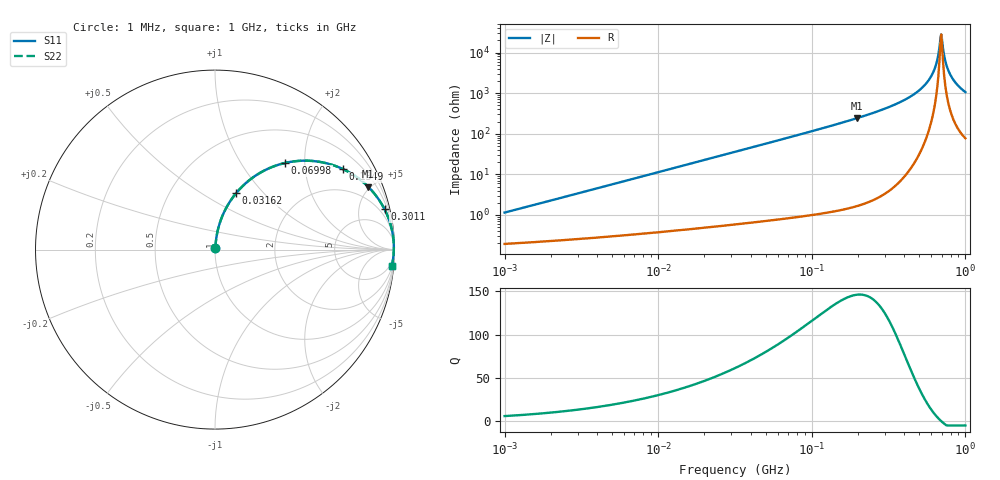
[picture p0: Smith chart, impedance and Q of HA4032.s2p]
# MHz S MA R 50
!Freq  MagS11  AngS11  MagS21  AngS21  MagS12  AngS12  MagS22  AngS22
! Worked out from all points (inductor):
!   801 points, 1 MHz to 1 GHz, reference 50 ohm
!   read as one part in series: L = 180 nH near 1.035 MHz
!   highest Q = 146 at 197.2 MHz (marker M1), where L = 196 nH
!   self-resonance near 689.8 MHz
!   S11 on the Smith chart (normalised r, x): 1 MHz: 1.00, +0.02; 31.62 MHz: 1.01, +0.72; 69.98 MHz: 1.02, +1.60; 134.9 MHz: 1.02, +3.17; 301.1 MHz: 1.07, +8.38; 1 GHz: 3, -21
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1  0.01145 79.6  0.998 -0.6  0.998 -0.6  0.01145 79.6
3.180534  0.03595 83.8  0.9968 -2.1  0.9968 -2.1  0.03595 83.8
10.02882  0.1124 81.7  0.99 -6.4  0.99 -6.4  0.1124 81.7
31.62278  0.3357 69.5  0.9365 -19.6  0.9365 -19.6  0.3357 69.5
31.89701  0.3383 69.3  0.9356 -19.8  0.9356 -19.8  0.3383 69.3
69.9842  0.6214 51.0  0.7771 -38.4  0.7771 -38.4  0.6214 51.0
100.5773  0.7547 40.5  0.6496 -49.0  0.6496 -49.0  0.7547 40.5
134.8963  0.8429 32.1  0.5317 -57.4  0.5317 -57.4  0.8429 32.1
197.2423  0.9223 22.3  0.3802 -67.3  0.3802 -67.3  0.9223 22.3
301.1272  0.9709 13.4  0.2316 -76.1  0.2316 -76.1  0.9709 13.4
317.1393  0.9747 12.4  0.2152 -77.1  0.2152 -77.1  0.9747 12.4
444.1197  0.9911 6.7  0.1169 -82.3  0.1169 -82.3  0.9911 6.7
555.9043  0.9958 3.3  0.05727 -84.2  0.05727 -84.2  0.9958 3.3
627.3357  0.9966 1.5  0.02639 -81.9  0.02639 -81.9  0.9966 1.5
649.3816  0.9966 1.0  0.01772 -78.6  0.01772 -78.6  0.9966 1.0
678.0317  0.9965 0.4  0.007339 -61.7  0.007339 -61.7  0.9965 0.4
695.825  0.9964 -0.0  0.003581 1.2  0.003581 1.2  0.9964 -0.0
714.0851  0.9962 -0.4  0.00761 60.2  0.00761 60.2  0.9962 -0.4
752.0557  0.9957 -1.1  0.02017 77.2  0.02017 77.2  0.9957 -1.1
798.9139  0.9949 -2.0  0.03539 80.6  0.03539 80.6  0.9949 -2.0
886.1352  0.9926 -3.5  0.06186 81.4  0.06186 81.4  0.9926 -3.5
1000  0.9888 -5.3  0.09337 80.5  0.09337 80.5  0.9888 -5.3
